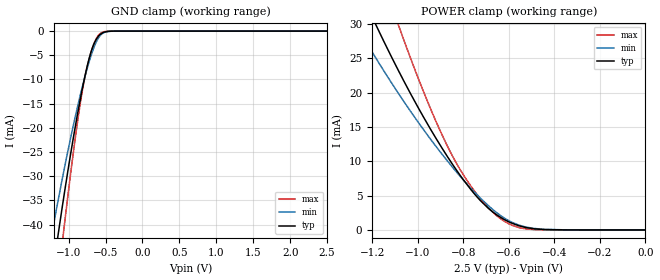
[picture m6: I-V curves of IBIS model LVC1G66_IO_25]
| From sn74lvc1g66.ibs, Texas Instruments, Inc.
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[Model]   LVC1G66_IO_25
Model_type  Terminator
| variable   typ   min   max
C_comp   6.85pF   1.30pF   17.24pF
| C_tri-state   6.85pF   1.30pF   17.24pF
[Temperature Range]   40   100   -40
| Ambient temperature   25   85   -40
[Voltage range]   2.5   2.3   2.7
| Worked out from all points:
|   GND clamp passes 1 mA (typ) near -0.59 V on its own axis
|   POWER clamp passes 1 mA (typ) near -0.59 V on its own axis
[GND Clamp]
| LVC1G66_IO_25
|   Voltage   I(typ)   I(min)   I(max)
-5.5V     -642.4mA   -532.1mA   -759.1mA
-1.235V   -51.96mA   -42.61mA   -64.15mA
-1.19V    -47.13mA   -38.88mA   -57.88mA
-1.145V   -42.4mA    -35.23mA   -51.73mA
-1.105V   -38.28mA   -32.06mA   -46.36mA
-1.065V   -34.27mA   -28.96mA   -41.11mA
-905mV    -19.35mA   -17.38mA   -21.59mA
-800mV    -10.87mA   -10.66mA   -11.16mA
-680mV    -3.569mA   -4.342mA   -3.58mA
-565mV    -610.2uA   -807.1uA   -430uA
-345mV    -2.421uA   -4.134uA   -261.5nA
2.5V      115.5pA    223nA      26.45pA
[POWER Clamp]
| LVC1G66_IO_25
|   Voltage   I(typ)   I(min)   I(max)
-5.5V     595.9mA    479.3mA    795.3mA
-1.275V   36.48mA    30.09mA    49.14mA
-1.24V    33.9mA     28.11mA    45.37mA
-1.18V    29.62mA    24.83mA    39.14mA
-1.09V    23.55mA    20.16mA    30.35mA
-1.06V    21.63mA    18.67mA    27.57mA
-945mV    14.75mA    13.28mA    17.76mA
-850mV    9.701mA    9.249mA    10.93mA
-745mV    5.021mA    5.315mA    5.404mA
-655mV    2.248mA    2.569mA    2.134mA
-490mV    173.3uA    227.1uA    56.83uA
-95.1fV   115.5pA    794.7pA    31.01pA
